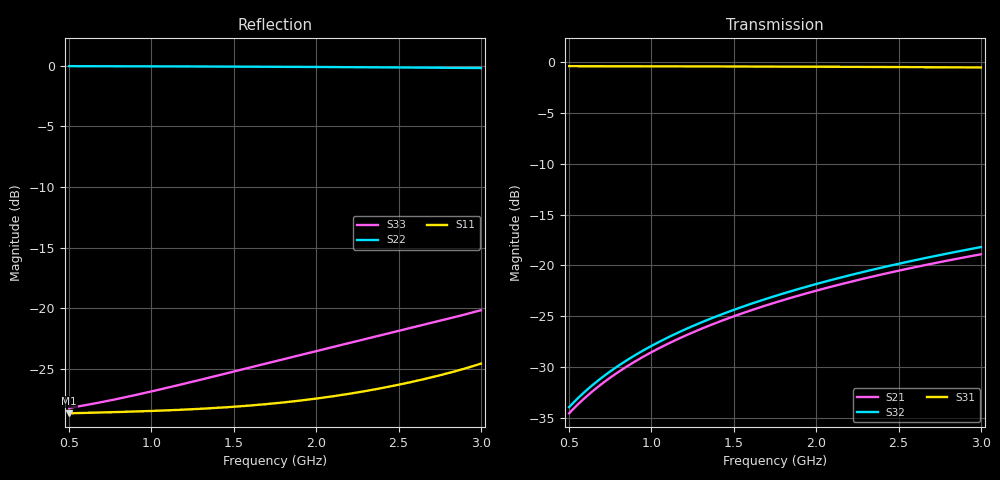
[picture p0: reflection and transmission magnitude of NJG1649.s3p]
! port1:P1 port2:P2 port3:PC
# hz S ma R 50
! 3 Port Network Data from SP1.SP block
! freq  magS11  angS11  magS12  angS12  magS13  angS13
!  magS21  angS21
!  magS22  angS22  magS23  angS23
!  magS31  angS31  magS32  angS32
!  magS33  angS33
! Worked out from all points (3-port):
!   251 points, 500 MHz to 3 GHz, reference 50 ohm
!   strongest paths, dB at 500 MHz, 1.12 GHz, 1.75 GHz, 2.38 GHz, 3 GHz:
!     S31: -0.4, -0.4, -0.4, -0.4, -0.5
!     S32: -34.0, -27.0, -23.0, -20.3, -18.2
!     S21: -34.6, -27.6, -23.7, -21.0, -18.9
!   lowest |S11| = -28.7 dB at 500 MHz (marker M1), VSWR 1.08, Z = 53.6 - j1.3 ohm
!   |S11| at or under -10 dB: start of sweep to end of sweep
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5e8  0.03688 -19.2  0.01865 80.1  0.9591 -6.4
     0.01865 80.1  0.9972 -6.3  0.02001 81.3
     0.9591 -6.4  0.02001 81.3  0.03881 -24.2
6e8  0.03703 -23.1  0.02238 79.1  0.9588 -7.7
     0.02238 79.1  0.997 -7.5  0.02401 80.5
     0.9588 -7.7  0.02401 80.5  0.03986 -28.7
7.2e8  0.03721 -27.8  0.02686 77.7  0.9585 -9.3
       0.02686 77.7  0.9966 -9.0  0.02882 79.3
       0.9585 -9.3  0.02882 79.3  0.04131 -33.8
8.5e8  0.03743 -32.9  0.03171 76.0  0.9581 -10.9
       0.03171 76.0  0.9962 -10.7  0.03404 78.0
       0.9581 -10.9  0.03404 78.0  0.04309 -39.0
1e9  0.03772 -38.9  0.03732 74.0  0.9576 -12.9
     0.03732 74.0  0.9957 -12.6  0.04008 76.3
     0.9576 -12.9  0.04008 76.3  0.04541 -44.8
1.34e9  0.03863 -52.8  0.05007 69.3  0.9564 -17.3
        0.05007 69.3  0.9941 -16.9  0.05384 72.3
        0.9564 -17.3  0.05384 72.3  0.05155 -56.4
1.75e9  0.04056 -70.2  0.06553 63.4  0.9545 -22.6
        0.06553 63.4  0.9916 -22.1  0.07059 67.4
        0.9545 -22.6  0.07059 67.4  0.06043 -68.4
2.42e9  0.04718 -99.1  0.09104 53.4  0.9503 -31.4
        0.09104 53.4  0.986 -30.6  0.09843 58.9
        0.9503 -31.4  0.09843 58.9  0.07817 -84.8
2.73e9  0.05249 -112.0  0.1029 48.7  0.9478 -35.6
        0.1029 48.7  0.9828 -34.6  0.1115 54.8
        0.9478 -35.6  0.1115 54.8  0.08803 -91.7
3e9  0.05913 -122.9  0.1134 44.4  0.9451 -39.2
     0.1134 44.4  0.9797 -38.2  0.1231 51.2
     0.9451 -39.2  0.1231 51.2  0.09821 -97.7
